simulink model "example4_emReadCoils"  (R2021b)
settings: Solver=FixedStepAuto  StartTime=0  StopTime=inf  FixedStep=0.5  RelTol=1e-3  EnableMultiTasking=on
undefined symbols (not defined in the file or in its folder): based, classic, dsPic33, MCC, Microchip, PIC24
libraries: emMBSlaveLib x2, embeddedCreatorLib x1

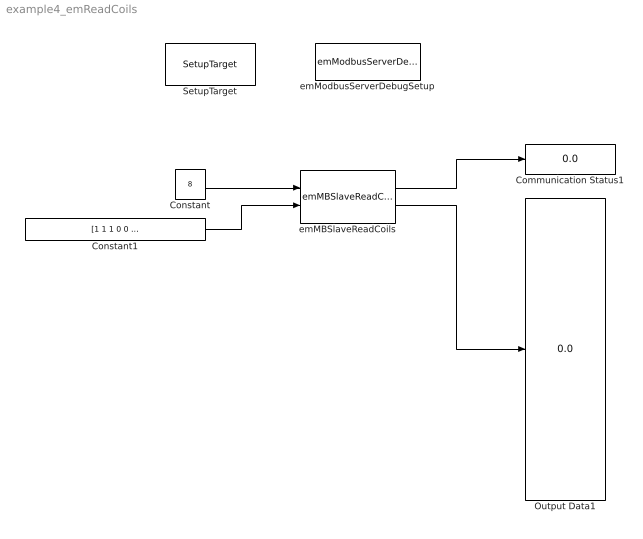
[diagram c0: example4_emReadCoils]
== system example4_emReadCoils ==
  Communication Status1 : Display
  Constant : Constant  Value=8  OutDataTypeStr=uint16
  Constant1 : Constant  Value=[1 1 1 0 0 0 1 1 1 0 0 0 1 1 1 1 1]  OutDataTypeStr=boolean
  Output Data1 : Display
  SetupTarget : embeddedCreatorLib/SetupTarget  Tag=SetupTarget  Priority=0  c_platform=Microchip PIC24/dsPic33 based on MCC classic  c_debug=on
  emMBSlaveReadCoils : emMBSlaveLib/emMBSlaveReadCoils  c_ServerID=1  c_minAdr=8  c_RegQTY=18  c_sampleTime=-1
  emModbusServerDebugSetup : emMBSlaveLib/emModbusServerDebugSetup  Tag=emModbusSlaveSetup  c_objID=0  c_uartNo=2  c_baudrate=19200  c_serverID=1  c_baudrate4PC=19200  c_forceLongerSpace=on  c_holdingRegsQTY=0  c_minHoldingAddr=789  c_inputRegsQTY=0  c_minInputRegAddr=1  c_coilRegsQTY=18  c_minCoilAddr=8  c_discreteRegsQTY=0  c_minDiscreteAddr=8  c_enableDebug=on  c_breakpointMaxQTY=100  c_probeMaxWordQTY=200  c_emWaitQTY=0  g_COMPortNo=COM5  c_Name_method=By physical port name and bit number  c_PortName=B  c_BitNo=11  c_TxEnable485="\"LATBbits.LATB11\""  c_TxEnable485Polarity=on
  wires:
  Constant/1 -> emMBSlaveReadCoils/1
  emMBSlaveReadCoils/1 -> Communication Status1/1
  emMBSlaveReadCoils/2 -> Output Data1/1
  Constant1/1 -> emMBSlaveReadCoils/2
